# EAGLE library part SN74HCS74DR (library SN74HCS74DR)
Flip-Flops Schmitt-trigger input dual D-type positive-edge-triggered flip-flops w/ clear and preset 14-SOIC -40 to 125 Source: Datasheet
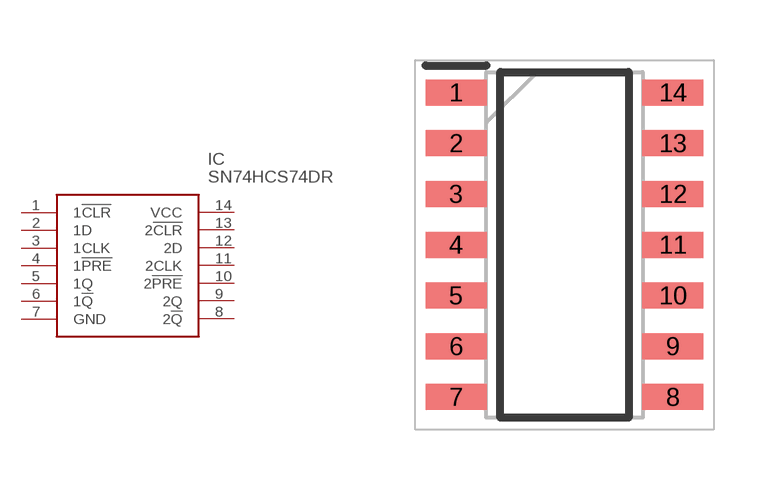
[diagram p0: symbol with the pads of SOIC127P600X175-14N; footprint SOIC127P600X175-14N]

Designator prefix IC

## SN74HCS74DR (Description: Flip-Flops Schmitt-trigger input dual D-type positive-edge-triggered flip-flops w/ clear and preset 14-SOIC -40 to 125; Height: 1.75mm; Manufacturer_Name: Texas Instruments; Manufacturer_Part_Number: SN74HCS74DR; Mouser_Part_Number: 595-SN74HCS74DR; Mouser_Price-Stock: https://www.mouser.co.uk/ProductDetail/Texas-Instruments/SN74HCS74DR?qs=TiOZkKH1s2QvGxo75w4r5Q%3D%3D)  [SOIC127P600X175-14N]
1  1!CLR
2  1D
3  1CLK
4  1!PRE
5  1Q
6  1!Q
7  GND
8  2!Q
9  2Q
10  2!PRE
11  2CLK
12  2D
13  2!CLR
14  VCC

## Footprint SOIC127P600X175-14N (pad centres in mm)
D (-R-PDSO-G14).
smd 1.525 x 0.65: 1 -2.712,3.81; 2 -2.712,2.54; 3 -2.712,1.27; 4 -2.712,0; 5 -2.712,-1.27; 6 -2.712,-2.54; 7 -2.712,-3.81; 8 2.712,-3.81; 9 2.712,-2.54; 10 2.712,-1.27; 11 2.712,0; 12 2.712,1.27; 13 2.712,2.54; 14 2.712,3.81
